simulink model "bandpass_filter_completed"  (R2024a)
settings: Solver=VariableStepDiscrete  StartTime=0.0  StopTime=inf  RelTol=1e-3  EnableMultiTasking=on
undefined symbols (not defined in the file or in its folder): code, Convert_config, Evaluation, ffva1156, gateway_in_config, gateway_out_config, hex2dec, KCU105, Kintex, Platform, Register_config, rodinimport_config, sysgen, UltraScale, xcku040, xfirv7_2_cmodel, xlfda_numerator
libraries: hdlBasic x5, dspsrcs4 x1, dspobslib x1, vmcUtilities x1, hdlUtilities x1, hdlDSPIP x1

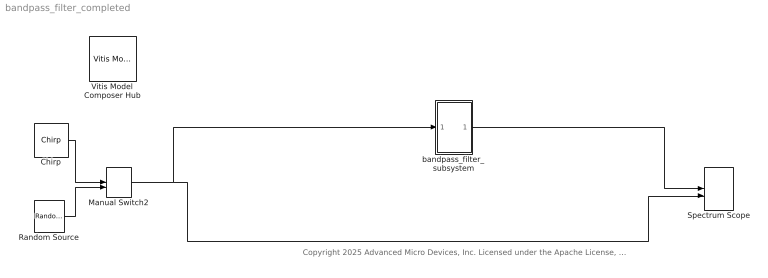
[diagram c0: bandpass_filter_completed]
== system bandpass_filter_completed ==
  note: Copyright 2025 Advanced Micro Devices, Inc. Licensed under the Apache License, Version 2.0 (the "License"); you may not use this file except in compliance with the License. You may obtain a copy of the License at http://www.apache.org/licenses/LICENSE-2.0 Unless required by applicable law or agreed to in writing, software distributed under the License is distributed on an "AS IS" BASIS, WITHOUT WARRANTIES OR CONDITIONS OF ANY KIND, either express or implied. See the License for the specific language governing permissions and limitations under the License.
  Chirp : dspsrcs4/Chirp  sweep=Swept cosine  mode=Bidirectional  f0=300000  f1=800000  t1=0.01  Tsweep=0.01  phase=0  Ts=1/3000000  spf=1  datatype=double  OutputFrames=on
  Manual Switch2 : ManualSwitch
  Random Source : dspobslib/Random Source  SrcType=Uniform  NormMethod=Ziggurat  CltLength=12  MinVal=-1  MaxVal=1  MeanVal=0  VarVal=1  RepMode=Not repeatable  rawSeed=1  IsInherit=off  SampMode=Discrete  SampTime=1/3000000  SampFrame=1  DataType=Double  OutComplex=Real  OutputFrames=on
  Spectrum Scope : SpectrumAnalyzer  NumInputPorts=2  WindowPosition=[486.000000,116.000000,1384.000000,667.000000,]  ScopeFrameLocation=window  Method=Welch  SampleRate=3000000  PlotAsTwoSidedSpectrum=off  AxesScaling=Manual  FrequencyResolutionMethod=Window length  RBWSource=Property  RBW=8789.0625  WindowLength=512  FFTLengthSource=Property  FFTLength=512  Span=1500000  CenterFrequency=750000  StartFrequency=0  StopFrequency=1500000  OverlapPercent=50  AveragingMethod=Running  SpectralAverages=2  YLabel=Magnitude-squared  YLimits=[-146,44]  AllowFFTLengthLessThanSamplesPerUpdate=on  SegLen=512
  Vitis Model Composer Hub : vmcUtilities/Vitis Model Composer Hub  Tag=genX  CodeGeneration=off  SubsystemName=bandpass_filter  StartColumn=1  NumberOfColumns=1  TargetDirectory=./code  exportDesign=off  analyzeDesign=off  validateDesignOnHw=off  ExportType=HDL  IpVendor=xilinx.com  IpLibrary=hls  IpVersion=1.0  IpHWLanguage=Verilog  AieCompilerOptions={}  AieSimulatorOptions={}  CreateTestbench=off  TestbenchStackSize=10  RunRtlSim=off  RunCSim=off  RunAieSim=off  AieSimTimeout=50000  RunAieSimProfiling=off  LaunchVitisAnalyzer=off  PlotOutput=off  RunX86Sim=off  X86SimTimeout=10  GenHwImage=off  GenLibadfXo=off  GenHwValidationCode=off  PlatformType=Not Specified  HwSystemType=Baremetal  HwValidationTarget=hw  ProjDevice=Kintex-UltraScale KCU105 Evaluation Platform (xcku040-ffva1156-2-e)  ProjDevicePart=xcku040-ffva1156-2-e  AIEType=None  SamplePeriod=-1  ClockFrequency=200  DataPathParallelism=1  xilinxfamily=kintexu  part=xcku040  speed=-2-e  package=ffva1156  directory=./netlist_hwcs/ip/bandpass_filter/src  testbench=off  incr_netlist=off  synthesis_tool=Vivado  clock_wrapper=Clock Enables  dbl_ovrd=According to Block Masks  dcm_input_clock_period=10  sysclk_period=10  simulink_period=1/(3*3000000)  eval_field=0  IPInfoJsonString="{\"HDLSubsystem\":{\"SubsystemName\":\"bandpass_filter\",\"IPName\":\"bandpass_filter\",\"IPLibrary\":\"VMC\",\"IPVendor\":\"User Company\",\"IPVersion\":\"1.0\",\"TargetDirectory\":\"./netlist_hwcs\",\"SubsystemDir\":\"./netlist_hwcs/ip/bandpass_filter\"}}"  LogFileName=''  NThreads=4
  bandpass_filter_subsystem : Subsystem
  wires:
  Chirp/1 -> Manual Switch2/1
  Random Source/1 -> Manual Switch2/2
  Manual Switch2/1 -> bandpass_filter_subsystem/1(In1), Spectrum Scope/2
  bandpass_filter_subsystem/1(Out1) -> Spectrum Scope/1

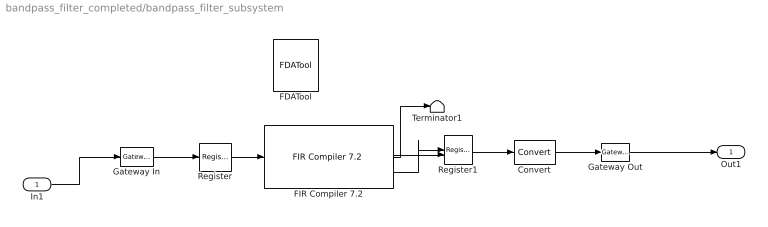
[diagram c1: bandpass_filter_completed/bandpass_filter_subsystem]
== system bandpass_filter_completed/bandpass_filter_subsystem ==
  In1 : Inport
  Convert : hdlBasic/Convert  gui_display_data_type=Fixed-point  arith_type=Signed (2's comp)  n_bits=8  bin_pt=6  float_type=Single  exp_bits=8  fraction_bits=24  quantization=Truncate  overflow=Wrap  en=off  latency=1  pipeline=off  XmcBlockStatus=1  maskContainerNames=group2  block_type=convert  block_config=sysgen:Convert_config  block_width=595  block_height=885
  FDATool : hdlUtilities/FDATool  block_type=fdatool
  FIR Compiler 7.2 : hdlDSPIP/FIR Compiler 7.2   coefficientvector=xlfda_numerator('FDATool')  coefficient_sets=1  coefficient_reload=off  filter_type=Single_Rate  rate_change_type=Integer  interpolation_rate=1  decimation_rate=1  zero_pack_factor=1  channel_sequence=Basic  number_channels=1  pattern_list='P4-0,P4-1,P4-2,P4-3,P4-4'  number_paths=1  ratespecification=Maximum_Possible  sampleperiod=3  hardwareoversamplingrate=1  coefficient_sign=Signed  quantization=Maximize_Dynamic_Range  coefficient_width=12  bestprecision=on  coefficient_fractional_bits=13  coefficient_structure=Inferred  output_rounding_mode=Full_Precision  output_width=31  filter_architecture=Systolic_Multiply_Accumulate  optimization_goal=Area  optimization_list='None'  data_buffer_type=Automatic  coefficient_buffer_type=Automatic  input_buffer_type=Automatic  output_buffer_type=Automatic  preference_for_other_storage=Automatic  multi_column_support=Automatic  columnconfig='46'  inter_column_pipe_length=4  data_has_tlast=Not_Required  m_data_has_tready=off  s_data_has_fifo=off  s_data_has_tuser=Not_Required  m_data_has_tuser=Not_Required  s_config_sync_mode=On_Vector  s_config_method=Single  num_reload_slots=1  has_aclken=off  has_aresetn=off  reset_data_vector=on  trim_axipin_name=on  simulation_type=hybrid_sim  simulation_model=sysgen:xfirv7_2_cmodel  data_path_portlist={ 's_axis_data_tdata', 'm_axis_data_tdata' }  passband_min=0.0  passband_max=0.5  stopband_min=0.5  stopband_max=1.0  filter_selection=1  gui_behaviour='Sysgen_GUI'  data_sign=Signed  data_width=16  data_fractional_bits=0  data_tuser_width=1  wrapper_available=true  ip_wrap_arbitrary_binary_point=true  ip_name=FIR Compiler  ip_version=7.2  dsptool_ready=true  ipcore_usecache=true  ipcore_useipmodelcache=true  port_translation_map={ 'aclken' => 'en', 'aresetn' => 'rst' }  run_core_at_system_period=true  ipcore_xco_need_fpga_part=true  ipcore_fpga_part=[]  XmcBlockStatus=1  maskContainerNames=tabcontainer1  block_type=fir_compiler_v7_2  block_config=sysgen:rodinimport_config  block_width=820  block_height=600
  Gateway In : hdlBasic/Gateway In  gui_display_data_type=Fixed-point  arith_type=Signed (2's comp)  n_bits=8  bin_pt=6  preci_type=Single  exp_width=8  frac_width=24  rows=1  columns=1  quantization="Round  (unbiased: +/- Inf)"  overflow=Saturate  period=1/3000000  UseAsADC=off  ADCChannel='1'  interface=None  automatic_assignment=on  address_offset=hex2dec('00')  intf_name=''  intf_description=''  default_value=0  timing_constraint=None  locs_specified=off  LOCs={}  io_standard={}  inherit_from_input=off  hdl_port=on  XmcBlockStatus=1  maskContainerNames=group4  block_type=gatewayin  block_config=sysgen:gateway_in_config  block_width_w=590  block_height_w=620  block_width=640  block_height=850
  Gateway Out : hdlBasic/Gateway Out  inherit_from_input=off  hdl_port=on  rows=1  columns=1  UseAsDAC=off  DACChannel='1'  interface=None  automatic_assignment=on  address_offset=hex2dec('00')  intf_name=''  intf_description=''  timing_constraint=None  locs_specified=off  LOCs={}  io_standard={}  XmcBlockStatus=1  maskContainerNames=group4  block_type=gatewayout  block_config=sysgen:gateway_out_config  block_width_w=590  block_height_w=620  block_width=620  block_height=750
  Register : hdlBasic/Register  init=0  rst=off  en=off  XmcBlockStatus=1  maskContainerNames=tabcontainer1  block_type=register  block_config=sysgen:Register_config
  Register1 : hdlBasic/Register  init=0  rst=off  en=on  XmcBlockStatus=1  maskContainerNames=tabcontainer1  block_type=register  block_config=sysgen:Register_config
  Terminator1 : Terminator
  Out1 : Outport
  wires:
  Register1/1 -> Convert/1
  FIR Compiler 7.2/2 -> Register1/2
  Register/1 -> FIR Compiler 7.2/1
  Gateway In/1 -> Register/1
  FIR Compiler 7.2/1 -> Terminator1/1
  Convert/1 -> Gateway Out/1
  FIR Compiler 7.2/3 -> Register1/1
  Gateway Out/1 -> Out1/1
  In1/1 -> Gateway In/1
